ORGANIZATION_BLOCK MAIN:OB1
TITLE=Cancello elettrico automatico
//Simulatore: 09
//Versione: 1.0
//Data: 18/07/2001
//------------ Descrizione dell'impianto --------------------
//L'apertura e la chiusura di un cancello sono gestite dal
//motore M1 protetto dal relè termico FR.
//La posizione del cancello viene rilevata mediante due
//finecorsa SQ1 (cancello aperto) SQ2 (cancello chiuso).
//Per la sicurezza antiinfortunistica sono previste:
// - una fotocellula B che rileva l'interposizione fra
//   proiettore e ricevitore,
// - una costa pneumatica, posta nella parte fissa del
//   cancello che interviene nel caso di un'azione di
//   esterna di opposizione al movimento di chiusura
//   del cancello.
//
//L'apertura del cancello viene comandata dal pulsante SB1
//o dal pulsante SB2 del radiocomando, il pulsante SB3 può
//arrestare in qualsiasi momento l'apertura o la chiusura
//del cancello.
//Una volta avviata e completata l'apertura il cancello
//resterà nella posizione aperto per un certo tempo quindi
//verrà richiuso automaticamente.
//Durante la richiusura se interviene una delle due sicurezze
//il cancello verrà forzato in riapertura.
//Il comando del cancello può essere effetuata anche con il
//selettore a chiave SB4 che nella posizione 2 effetua
//e nella posizione 1 la chiusura del cancello.
//
//La fase di movimentazione viene segnalata da un lampeggiatore
//HL4 (il lampeggio deve essere gestito dal PLC).
//Nel caso di intervento del termico FR il motore M1 verrà
//arrestato e la lampada HL2 segnalerà l'intervento della
//protezione.
//La lampada HL1 segnala invece lo stato ON-OFF del motore M1.
//

BEGIN
NETWORK 1 //Apertura cancello
//
LD I1.1 //P_SB1
O I1.2 //P_SB2
O I1.0 //S_SB4_2
ON I0.6 //SQ3
O I0.1 //B
O Q0.3 //Marker Apertura
A I0.5 //FR
AN I0.7 //S_SB4_1
AN Q0.2 //Marker Chiusura
A I0.0 //SQ1
A I1.3 //P_SB3
= Q0.3 //Marker apertura

NETWORK 2 //Temporizzatore apertura
//
LDN I0.0 //SQ1
A I0.5 //SQ2
TON T37 +50 //FR

//Marker Aperto
NETWORK 3 //Chiusura cancello
//
LD T37
O Q0.2 //Marker Chiusura
O I0.7 //S_SB4_1
AN Q0.3 //Marker Apertura
AN I1.0 //S_SB4_2
A I0.6 //SQ3
A I0.2 //SQ2
A I0.5 //FR
AN I0.1 //B
A I1.3 //P_SB3
= Q0.2 //Marker Chiusura
= Q0.0

NETWORK 4 //Segnalazione Ciclo ON
//
LD I0.2 //Marker Apertura
= Q0.6 //Marker Chiusura
//Marker Aperto
//HL3
NETWORK 5 //Lampeggio Lampada Movimento
//
LD SM0.5 //
A Q0.6 //HL3
= Q0.1 //HL4

NETWORK 6 //Segnalazione relè termico scattato
//
LDN I0.5 //FR
= Q0.5 //HL2

NETWORK 7 //Segnalazione Motore ON
//
LD Q0.2 //KM1
O Q0.3 //KM2
= Q0.4 //HL1

END_ORGANIZATION_BLOCK

